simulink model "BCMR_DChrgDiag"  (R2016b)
settings: Solver=FixedStepDiscrete  StartTime=0.0  StopTime=10  FixedStep=0.01  RelTol=1e-3  EnableMultiTasking=on
undefined symbols (not defined in the file or in its folder): BCMR_bDChrgStopCActiveSw_C, BCMR_cntDChrgTCnntMax_C, BCMR_cntIsoFltTrigger_CW, BCMR_EVCCDiagccSw_C, BCMR_EVCCDiagSw_C, BCMR_G1E0PlatformSwDiag_C, BCMR_H1U0PlatformSwDiag_C, BCMR_iDcChrgDiffOvrCurr_C, BCMR_iDcChrgLowTempDiffOvrCurrMody_C, BCMR_iDcChrgLowTempOvrCurrCutOff_C, BCMR_iDcChrgLowTempOvrCurrHeal_C, BCMR_iDcChrgOvrCurr_C, BCMR_iDcChrgOvrVolt_C, BCMR_iDChrgCurrDiagLmt_C, BCMR_iDChrgCutOffVoltOvrCurrDet_C, BCMR_iDChrgCutOffVoltOvrCurrHeal_C, BCMR_kWaveFltFactor_C, BCMR_stCCSTimeout_C, BCMR_stCHMTimeout_C, BCMR_stCMLTimeout_C, BCMR_stCRMAATimeout_C, BCMR_stCROAATimeout_C, BCMR_stCROTimeout_C, BCMR_stCSDTimeout1_C, BCMR_stCSDTimeout2_C, BCMR_stCSTTimeout_C, BCMR_stCurrDwnTimeout_C, BCMR_stHvOnTimeout_C, BCMR_stNoTimeout_C, BCMR_stParaMish_C, BCMR_tBattLowTempDiagTempThrd_C, BCMR_tDcChrgIntfTempDiffLmt_C, BCMR_tDcChrgIntfTempLmt_C, BCMR_tiDChrgDetDiagDebs_C, BCMR_tiDChrgDetSec_C, BCMR_tiDChrgDiagBase_C, BCMR_tiDChrgHealDiagDebs_C, BCMR_tiDChrgIntfTempDwnLmt_C, BCMR_tiDChrgLowTOvrCurrDet_C, BCMR_tiDChrgLowTOvrCurrHeal_C, BCMR_tiDChrgMishCurrDetDiagDebs_C, BCMR_tiDChrgOvrCellVolt_C, BCMR_tiDChrgOvrSafeCellVoltDet_C, BCMR_tiDChrgVoltFltDetDebs_C, BCMR_tiDChrgVoltFltHealDebs_C, BCMR_uCC2ChkDiffDet_C, BCMR_uCC2ChkDiffHeal_C, BCMR_uCC2VoltHighDet_C, BCMR_uCC2VoltHighHeal_C, BCMR_uCC2VoltLowDet_C, BCMR_uCC2VoltLowHeal_C, BCMR_uDChrgHighTempDet_C, BCMR_uDChrgHighTempHeal_C, BCMR_uDChrgLowTempDet_C, BCMR_uDChrgLowTempHeal_C, BCMR_uDChrgOvrCellVoltDet_C, BCMR_uDChrgOvrCellVoltHeal_C, BCMR_uDChrgOvrSafeCellVoltDet_C, BCMR_uDChrgOvrSafeCellVoltHeal_C, bin2dec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
libraries: simulink x291
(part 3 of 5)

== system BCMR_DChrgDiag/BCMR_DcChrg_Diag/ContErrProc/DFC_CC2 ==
  BCMR_bDcOutputContErrDet : Inport
  BCMR_bDcOutputContErrHeal : Inport  Port=2
  BCMR_bCC2VolttLowErrDet : Inport  Port=3
  BCMR_bCC2VoltLowErrHeal : Inport  Port=4
  BCMR_bCC2VoltHighErrDet : Inport  Port=5
  BCMR_bCC2VoltHighErrHeal : Inport  Port=6
  Bitwise Operator9 : simulink/Logic and Bit Operations/Bitwise Operator  logicop=AND  UseBitMask=on  BitMask=bin2dec('00011000')  BitMaskRealWorld=Stored Integer
  Compare To Constant3 : simulink/Logic and Bit Operations/Compare To Constant  relop===  const=24  OutDataTypeStr=boolean
  DSM_ReportCheckSelfHeal : Subsystem  TreatAsAtomicUnit=on  RTWFcnName=DSM_ReportCheck  RTWFileName=SrvLib
  Data Store Read2 : DataStoreRead  DataStoreName=DFC_CC2Chk
  Data Store Read3 : DataStoreRead  DataStoreName=DFC_CC2Chk
  Data Store Write1 : DataStoreWrite  DataStoreName=DFC_CC2Chk
  Data Type Conversion1 : DataTypeConversion  OutDataTypeStr=uint8
  Logical Operator1 : Logic  Operator=OR  Inputs=3  AllPortsSameDT=off  OutDataTypeStr=boolean
  Logical Operator2 : Logic  Inputs=3  AllPortsSameDT=off  OutDataTypeStr=boolean
  BCMR_stCC2ChkVoltErr : Outport  OutputWhenDisabled=reset  InitialOutput=[0]
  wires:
  Compare To Constant3/1 -> Data Type Conversion1/1
  Bitwise Operator9/1 -> Compare To Constant3/1
  Logical Operator1/1 -> DSM_ReportCheckSelfHeal/2(Err)
  Logical Operator2/1 -> DSM_ReportCheckSelfHeal/3(Heal)
  DSM_ReportCheckSelfHeal/1(Dfc_id) -> Data Store Write1/1
  Data Store Read2/1 -> DSM_ReportCheckSelfHeal/1(Dfc_id_nv)
  Data Store Read3/1 -> Bitwise Operator9/1
  Data Type Conversion1/1 -> BCMR_stCC2ChkVoltErr/1  "BCMR_stCC2ChkVoltErr"
  BCMR_bCC2VoltHighErrHeal/1 -> Logical Operator2/3
  BCMR_bCC2VoltLowErrHeal/1 -> Logical Operator2/2
  BCMR_bDcOutputContErrHeal/1 -> Logical Operator2/1
  BCMR_bCC2VoltHighErrDet/1 -> Logical Operator1/3
  BCMR_bCC2VolttLowErrDet/1 -> Logical Operator1/2
  BCMR_bDcOutputContErrDet/1 -> Logical Operator1/1

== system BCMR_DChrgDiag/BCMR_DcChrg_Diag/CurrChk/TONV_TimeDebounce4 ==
  note: Turn On Delay Time Deboune
  T : Inport
  u : Inport  Port=2
  dT : Inport  Port=3
  Add : Sum
  Constant1 : Constant  Value=0  OutDataTypeStr=uint8
  Constant2 : Constant  OutDataTypeStr=uint8
  Constant3 : Constant  Value=0  OutDataTypeStr=single
  Delay : Delay  DelayLength=1  InitialCondition=0
  MinMax : MinMax  Inputs=2
  Product : Product  OutMin=[0]  OutMax=[65535]  OutDataTypeStr=single
  Relational Operator : RelationalOperator  OutDataTypeStr=boolean  RndMeth=Simplest
  Switch : Switch  Criteria=u2 ~= 0
  Switch1 : Switch  Criteria=u2 ~= 0
  y : Outport
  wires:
  u/1 -> Switch1/2, Switch/2
  Switch/1 -> Product/1
  dT/1 -> Switch1/1
  Constant3/1 -> Switch1/3
  Constant2/1 -> Switch/1
  Constant1/1 -> Switch/3
  Add/1 -> Product/2
  Product/1 -> Relational Operator/1, Delay/1
  Switch1/1 -> Add/1
  Delay/1 -> MinMax/2
  Relational Operator/1 -> y/1
  T/1 -> Relational Operator/2, MinMax/1
  MinMax/1 -> Add/2

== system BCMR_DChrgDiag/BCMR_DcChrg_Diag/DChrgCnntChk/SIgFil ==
  u : Inport
  Constant4 : Constant  Value=0  OutDataTypeStr=boolean
  Delay1 : Delay  DelayLength=1  InitialCondition=0
  Filter : Subsystem
  Switch4 : Switch  Criteria=u2 ~= 0
  Unit Delay1 : UnitDelay  InitialCondition=1  SampleTime=-1
  y : Outport
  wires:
  Delay1/1 -> Filter/2(In2)
  u/1 -> Filter/1(In1), Switch4/1
  Unit Delay1/1 -> Switch4/2
  Constant4/1 -> Unit Delay1/1
  Filter/1(Out) -> Switch4/3
  Switch4/1 -> y/1, Delay1/1

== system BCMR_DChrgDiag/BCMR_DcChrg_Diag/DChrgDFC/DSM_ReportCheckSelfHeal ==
  note: Fault report to diagnostic management system
  Dfc_id_nv : Inport  OutDataTypeStr=uint8
  Err : Inport  Port=2
  Heal : Inport  Port=3
  Bit Clear1 : simulink/Logic and Bit Operations/Bit Clear  iBit=4
  Bit Clear2 : simulink/Logic and Bit Operations/Bit Clear  iBit=3
  Bit Set : simulink/Logic and Bit Operations/Bit Set  iBit=4
  Bit Set1 : simulink/Logic and Bit Operations/Bit Set  iBit=3
  Bit Set2 : simulink/Logic and Bit Operations/Bit Set  iBit=3
  Bit Set4 : simulink/Logic and Bit Operations/Bit Set  iBit=7
  Constant1 : Constant  Value=0  OutDataTypeStr=uint8
  Constant7 : Constant  Value=0  OutDataTypeStr=boolean
  Delay2 : Delay  DelayLength=1  InitialCondition=1
  Delay3 : Delay  DelayLength=1  InitialCondition=0
  Logical Operator : Logic  Operator=OR  AllPortsSameDT=off  OutDataTypeStr=boolean
  Switch{1..4} (4 alike) : Switch  Criteria=u2 ~= 0
  Dfc_id : Outport  OutDataTypeStr=uint8
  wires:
  Dfc_id_nv/1 -> Bit Clear2/1, Bit Set4/1, Bit Clear1/1
  Bit Set4/1 -> Bit Set/1
  Constant7/1 -> Delay2/1
  Delay2/1 -> Switch2/2
  Switch3/1 -> Switch2/3
  Bit Clear2/1 -> Switch2/1
  Switch2/1 -> Delay3/1, Switch1/1
  Bit Set1/1 -> Switch3/1
  Bit Set/1 -> Bit Set1/1
  Switch4/1 -> Switch3/3
  Err/1 -> Logical Operator/2, Switch3/2
  Bit Set2/1 -> Switch4/1
  Bit Clear1/1 -> Bit Set2/1
  Delay3/1 -> Switch4/3
  Heal/1 -> Logical Operator/1, Switch4/2
  Logical Operator/1 -> Switch1/2
  Constant1/1 -> Switch1/3
  Switch1/1 -> Dfc_id/1

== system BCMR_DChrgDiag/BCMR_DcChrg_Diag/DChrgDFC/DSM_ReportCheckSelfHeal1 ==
  note: Fault report to diagnostic management system
  Dfc_id_nv : Inport  OutDataTypeStr=uint8
  Err : Inport  Port=2
  Heal : Inport  Port=3
  Bit Clear1 : simulink/Logic and Bit Operations/Bit Clear  iBit=4
  Bit Clear2 : simulink/Logic and Bit Operations/Bit Clear  iBit=3
  Bit Set : simulink/Logic and Bit Operations/Bit Set  iBit=4
  Bit Set1 : simulink/Logic and Bit Operations/Bit Set  iBit=3
  Bit Set2 : simulink/Logic and Bit Operations/Bit Set  iBit=3
  Bit Set4 : simulink/Logic and Bit Operations/Bit Set  iBit=7
  Constant1 : Constant  Value=0  OutDataTypeStr=uint8
  Constant7 : Constant  Value=0  OutDataTypeStr=boolean
  Delay2 : Delay  DelayLength=1  InitialCondition=1
  Delay3 : Delay  DelayLength=1  InitialCondition=0
  Logical Operator : Logic  Operator=OR  AllPortsSameDT=off  OutDataTypeStr=boolean
  Switch{1..4} (4 alike) : Switch  Criteria=u2 ~= 0
  Dfc_id : Outport  OutDataTypeStr=uint8
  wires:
  Dfc_id_nv/1 -> Bit Clear2/1, Bit Set4/1, Bit Clear1/1
  Bit Set4/1 -> Bit Set/1
  Constant7/1 -> Delay2/1
  Delay2/1 -> Switch2/2
  Switch3/1 -> Switch2/3
  Bit Clear2/1 -> Switch2/1
  Switch2/1 -> Delay3/1, Switch1/1
  Bit Set1/1 -> Switch3/1
  Bit Set/1 -> Bit Set1/1
  Switch4/1 -> Switch3/3
  Err/1 -> Logical Operator/2, Switch3/2
  Bit Set2/1 -> Switch4/1
  Bit Clear1/1 -> Bit Set2/1
  Delay3/1 -> Switch4/3
  Heal/1 -> Logical Operator/1, Switch4/2
  Logical Operator/1 -> Switch1/2
  Constant1/1 -> Switch1/3
  Switch1/1 -> Dfc_id/1

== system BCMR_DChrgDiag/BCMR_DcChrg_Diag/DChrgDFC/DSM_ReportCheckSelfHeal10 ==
  note: Fault report to diagnostic management system
  Dfc_id_nv : Inport  OutDataTypeStr=uint8
  Err : Inport  Port=2
  Heal : Inport  Port=3
  Bit Clear1 : simulink/Logic and Bit Operations/Bit Clear  iBit=4
  Bit Clear2 : simulink/Logic and Bit Operations/Bit Clear  iBit=3
  Bit Set : simulink/Logic and Bit Operations/Bit Set  iBit=4
  Bit Set1 : simulink/Logic and Bit Operations/Bit Set  iBit=3
  Bit Set2 : simulink/Logic and Bit Operations/Bit Set  iBit=3
  Bit Set4 : simulink/Logic and Bit Operations/Bit Set  iBit=7
  Constant1 : Constant  Value=0  OutDataTypeStr=uint8
  Constant7 : Constant  Value=0  OutDataTypeStr=boolean
  Delay2 : Delay  DelayLength=1  InitialCondition=1
  Delay3 : Delay  DelayLength=1  InitialCondition=0
  Logical Operator : Logic  Operator=OR  AllPortsSameDT=off  OutDataTypeStr=boolean
  Switch{1..4} (4 alike) : Switch  Criteria=u2 ~= 0
  Dfc_id : Outport  OutDataTypeStr=uint8
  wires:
  Dfc_id_nv/1 -> Bit Clear2/1, Bit Set4/1, Bit Clear1/1
  Bit Set4/1 -> Bit Set/1
  Constant7/1 -> Delay2/1
  Delay2/1 -> Switch2/2
  Switch3/1 -> Switch2/3
  Bit Clear2/1 -> Switch2/1
  Switch2/1 -> Delay3/1, Switch1/1
  Bit Set1/1 -> Switch3/1
  Bit Set/1 -> Bit Set1/1
  Switch4/1 -> Switch3/3
  Err/1 -> Logical Operator/2, Switch3/2
  Bit Set2/1 -> Switch4/1
  Bit Clear1/1 -> Bit Set2/1
  Delay3/1 -> Switch4/3
  Heal/1 -> Logical Operator/1, Switch4/2
  Logical Operator/1 -> Switch1/2
  Constant1/1 -> Switch1/3
  Switch1/1 -> Dfc_id/1

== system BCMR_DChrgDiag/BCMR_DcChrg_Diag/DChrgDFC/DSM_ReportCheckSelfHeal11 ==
  note: Fault report to diagnostic management system
  Dfc_id_nv : Inport  OutDataTypeStr=uint8
  Err : Inport  Port=2
  Heal : Inport  Port=3
  Bit Clear1 : simulink/Logic and Bit Operations/Bit Clear  iBit=4
  Bit Clear2 : simulink/Logic and Bit Operations/Bit Clear  iBit=3
  Bit Set : simulink/Logic and Bit Operations/Bit Set  iBit=4
  Bit Set1 : simulink/Logic and Bit Operations/Bit Set  iBit=3
  Bit Set2 : simulink/Logic and Bit Operations/Bit Set  iBit=3
  Bit Set4 : simulink/Logic and Bit Operations/Bit Set  iBit=7
  Constant1 : Constant  Value=0  OutDataTypeStr=uint8
  Constant7 : Constant  Value=0  OutDataTypeStr=boolean
  Delay2 : Delay  DelayLength=1  InitialCondition=1
  Delay3 : Delay  DelayLength=1  InitialCondition=0
  Logical Operator : Logic  Operator=OR  AllPortsSameDT=off  OutDataTypeStr=boolean
  Switch{1..4} (4 alike) : Switch  Criteria=u2 ~= 0
  Dfc_id : Outport  OutDataTypeStr=uint8
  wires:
  Dfc_id_nv/1 -> Bit Clear2/1, Bit Set4/1, Bit Clear1/1
  Bit Set4/1 -> Bit Set/1
  Constant7/1 -> Delay2/1
  Delay2/1 -> Switch2/2
  Switch3/1 -> Switch2/3
  Bit Clear2/1 -> Switch2/1
  Switch2/1 -> Delay3/1, Switch1/1
  Bit Set1/1 -> Switch3/1
  Bit Set/1 -> Bit Set1/1
  Switch4/1 -> Switch3/3
  Err/1 -> Logical Operator/2, Switch3/2
  Bit Set2/1 -> Switch4/1
  Bit Clear1/1 -> Bit Set2/1
  Delay3/1 -> Switch4/3
  Heal/1 -> Logical Operator/1, Switch4/2
  Logical Operator/1 -> Switch1/2
  Constant1/1 -> Switch1/3
  Switch1/1 -> Dfc_id/1

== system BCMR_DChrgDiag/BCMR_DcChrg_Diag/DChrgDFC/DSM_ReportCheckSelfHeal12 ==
  note: Fault report to diagnostic management system
  Dfc_id_nv : Inport  OutDataTypeStr=uint8
  Err : Inport  Port=2
  Heal : Inport  Port=3
  Bit Clear1 : simulink/Logic and Bit Operations/Bit Clear  iBit=4
  Bit Clear2 : simulink/Logic and Bit Operations/Bit Clear  iBit=3
  Bit Set : simulink/Logic and Bit Operations/Bit Set  iBit=4
  Bit Set1 : simulink/Logic and Bit Operations/Bit Set  iBit=3
  Bit Set2 : simulink/Logic and Bit Operations/Bit Set  iBit=3
  Bit Set4 : simulink/Logic and Bit Operations/Bit Set  iBit=7
  Constant1 : Constant  Value=0  OutDataTypeStr=uint8
  Constant7 : Constant  Value=0  OutDataTypeStr=boolean
  Delay2 : Delay  DelayLength=1  InitialCondition=1
  Delay3 : Delay  DelayLength=1  InitialCondition=0
  Logical Operator : Logic  Operator=OR  AllPortsSameDT=off  OutDataTypeStr=boolean
  Switch{1..4} (4 alike) : Switch  Criteria=u2 ~= 0
  Dfc_id : Outport  OutDataTypeStr=uint8
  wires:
  Dfc_id_nv/1 -> Bit Clear2/1, Bit Set4/1, Bit Clear1/1
  Bit Set4/1 -> Bit Set/1
  Constant7/1 -> Delay2/1
  Delay2/1 -> Switch2/2
  Switch3/1 -> Switch2/3
  Bit Clear2/1 -> Switch2/1
  Switch2/1 -> Delay3/1, Switch1/1
  Bit Set1/1 -> Switch3/1
  Bit Set/1 -> Bit Set1/1
  Switch4/1 -> Switch3/3
  Err/1 -> Logical Operator/2, Switch3/2
  Bit Set2/1 -> Switch4/1
  Bit Clear1/1 -> Bit Set2/1
  Delay3/1 -> Switch4/3
  Heal/1 -> Logical Operator/1, Switch4/2
  Logical Operator/1 -> Switch1/2
  Constant1/1 -> Switch1/3
  Switch1/1 -> Dfc_id/1

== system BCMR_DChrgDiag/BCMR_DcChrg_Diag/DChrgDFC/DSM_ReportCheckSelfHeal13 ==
  note: Fault report to diagnostic management system
  Dfc_id_nv : Inport  OutDataTypeStr=uint8
  Err : Inport  Port=2
  Heal : Inport  Port=3
  Bit Clear1 : simulink/Logic and Bit Operations/Bit Clear  iBit=4
  Bit Clear2 : simulink/Logic and Bit Operations/Bit Clear  iBit=3
  Bit Set : simulink/Logic and Bit Operations/Bit Set  iBit=4
  Bit Set1 : simulink/Logic and Bit Operations/Bit Set  iBit=3
  Bit Set2 : simulink/Logic and Bit Operations/Bit Set  iBit=3
  Bit Set4 : simulink/Logic and Bit Operations/Bit Set  iBit=7
  Constant1 : Constant  Value=0  OutDataTypeStr=uint8
  Constant7 : Constant  Value=0  OutDataTypeStr=boolean
  Delay2 : Delay  DelayLength=1  InitialCondition=1
  Delay3 : Delay  DelayLength=1  InitialCondition=0
  Logical Operator : Logic  Operator=OR  AllPortsSameDT=off  OutDataTypeStr=boolean
  Switch{1..4} (4 alike) : Switch  Criteria=u2 ~= 0
  Dfc_id : Outport  OutDataTypeStr=uint8
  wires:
  Dfc_id_nv/1 -> Bit Clear2/1, Bit Set4/1, Bit Clear1/1
  Bit Set4/1 -> Bit Set/1
  Constant7/1 -> Delay2/1
  Delay2/1 -> Switch2/2
  Switch3/1 -> Switch2/3
  Bit Clear2/1 -> Switch2/1
  Switch2/1 -> Delay3/1, Switch1/1
  Bit Set1/1 -> Switch3/1
  Bit Set/1 -> Bit Set1/1
  Switch4/1 -> Switch3/3
  Err/1 -> Logical Operator/2, Switch3/2
  Bit Set2/1 -> Switch4/1
  Bit Clear1/1 -> Bit Set2/1
  Delay3/1 -> Switch4/3
  Heal/1 -> Logical Operator/1, Switch4/2
  Logical Operator/1 -> Switch1/2
  Constant1/1 -> Switch1/3
  Switch1/1 -> Dfc_id/1

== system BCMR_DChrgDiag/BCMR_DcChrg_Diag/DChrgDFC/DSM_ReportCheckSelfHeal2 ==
  note: Fault report to diagnostic management system
  Dfc_id_nv : Inport  OutDataTypeStr=uint8
  Err : Inport  Port=2
  Heal : Inport  Port=3
  Bit Clear1 : simulink/Logic and Bit Operations/Bit Clear  iBit=4
  Bit Clear2 : simulink/Logic and Bit Operations/Bit Clear  iBit=3
  Bit Set : simulink/Logic and Bit Operations/Bit Set  iBit=4
  Bit Set1 : simulink/Logic and Bit Operations/Bit Set  iBit=3
  Bit Set2 : simulink/Logic and Bit Operations/Bit Set  iBit=3
  Bit Set4 : simulink/Logic and Bit Operations/Bit Set  iBit=7
  Constant1 : Constant  Value=0  OutDataTypeStr=uint8
  Constant7 : Constant  Value=0  OutDataTypeStr=boolean
  Delay2 : Delay  DelayLength=1  InitialCondition=1
  Delay3 : Delay  DelayLength=1  InitialCondition=0
  Logical Operator : Logic  Operator=OR  AllPortsSameDT=off  OutDataTypeStr=boolean
  Switch{1..4} (4 alike) : Switch  Criteria=u2 ~= 0
  Dfc_id : Outport  OutDataTypeStr=uint8
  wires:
  Dfc_id_nv/1 -> Bit Clear2/1, Bit Set4/1, Bit Clear1/1
  Bit Set4/1 -> Bit Set/1
  Constant7/1 -> Delay2/1
  Delay2/1 -> Switch2/2
  Switch3/1 -> Switch2/3
  Bit Clear2/1 -> Switch2/1
  Switch2/1 -> Delay3/1, Switch1/1
  Bit Set1/1 -> Switch3/1
  Bit Set/1 -> Bit Set1/1
  Switch4/1 -> Switch3/3
  Err/1 -> Logical Operator/2, Switch3/2
  Bit Set2/1 -> Switch4/1
  Bit Clear1/1 -> Bit Set2/1
  Delay3/1 -> Switch4/3
  Heal/1 -> Logical Operator/1, Switch4/2
  Logical Operator/1 -> Switch1/2
  Constant1/1 -> Switch1/3
  Switch1/1 -> Dfc_id/1

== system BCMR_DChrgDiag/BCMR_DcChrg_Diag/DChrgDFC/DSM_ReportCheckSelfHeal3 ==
  note: Fault report to diagnostic management system
  Dfc_id_nv : Inport  OutDataTypeStr=uint8
  Err : Inport  Port=2
  Heal : Inport  Port=3
  Bit Clear1 : simulink/Logic and Bit Operations/Bit Clear  iBit=4
  Bit Clear2 : simulink/Logic and Bit Operations/Bit Clear  iBit=3
  Bit Set : simulink/Logic and Bit Operations/Bit Set  iBit=4
  Bit Set1 : simulink/Logic and Bit Operations/Bit Set  iBit=3
  Bit Set2 : simulink/Logic and Bit Operations/Bit Set  iBit=3
  Bit Set4 : simulink/Logic and Bit Operations/Bit Set  iBit=7
  Constant1 : Constant  Value=0  OutDataTypeStr=uint8
  Constant7 : Constant  Value=0  OutDataTypeStr=boolean
  Delay2 : Delay  DelayLength=1  InitialCondition=1
  Delay3 : Delay  DelayLength=1  InitialCondition=0
  Logical Operator : Logic  Operator=OR  AllPortsSameDT=off  OutDataTypeStr=boolean
  Switch{1..4} (4 alike) : Switch  Criteria=u2 ~= 0
  Dfc_id : Outport  OutDataTypeStr=uint8
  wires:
  Dfc_id_nv/1 -> Bit Clear2/1, Bit Set4/1, Bit Clear1/1
  Bit Set4/1 -> Bit Set/1
  Constant7/1 -> Delay2/1
  Delay2/1 -> Switch2/2
  Switch3/1 -> Switch2/3
  Bit Clear2/1 -> Switch2/1
  Switch2/1 -> Delay3/1, Switch1/1
  Bit Set1/1 -> Switch3/1
  Bit Set/1 -> Bit Set1/1
  Switch4/1 -> Switch3/3
  Err/1 -> Logical Operator/2, Switch3/2
  Bit Set2/1 -> Switch4/1
  Bit Clear1/1 -> Bit Set2/1
  Delay3/1 -> Switch4/3
  Heal/1 -> Logical Operator/1, Switch4/2
  Logical Operator/1 -> Switch1/2
  Constant1/1 -> Switch1/3
  Switch1/1 -> Dfc_id/1

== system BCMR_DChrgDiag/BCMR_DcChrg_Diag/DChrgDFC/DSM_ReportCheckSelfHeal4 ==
  note: Fault report to diagnostic management system
  Dfc_id_nv : Inport  OutDataTypeStr=uint8
  Err : Inport  Port=2
  Heal : Inport  Port=3
  Bit Clear1 : simulink/Logic and Bit Operations/Bit Clear  iBit=4
  Bit Clear2 : simulink/Logic and Bit Operations/Bit Clear  iBit=3
  Bit Set : simulink/Logic and Bit Operations/Bit Set  iBit=4
  Bit Set1 : simulink/Logic and Bit Operations/Bit Set  iBit=3
  Bit Set2 : simulink/Logic and Bit Operations/Bit Set  iBit=3
  Bit Set4 : simulink/Logic and Bit Operations/Bit Set  iBit=7
  Constant1 : Constant  Value=0  OutDataTypeStr=uint8
  Constant7 : Constant  Value=0  OutDataTypeStr=boolean
  Delay2 : Delay  DelayLength=1  InitialCondition=1
  Delay3 : Delay  DelayLength=1  InitialCondition=0
  Logical Operator : Logic  Operator=OR  AllPortsSameDT=off  OutDataTypeStr=boolean
  Switch{1..4} (4 alike) : Switch  Criteria=u2 ~= 0
  Dfc_id : Outport  OutDataTypeStr=uint8
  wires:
  Dfc_id_nv/1 -> Bit Clear2/1, Bit Set4/1, Bit Clear1/1
  Bit Set4/1 -> Bit Set/1
  Constant7/1 -> Delay2/1
  Delay2/1 -> Switch2/2
  Switch3/1 -> Switch2/3
  Bit Clear2/1 -> Switch2/1
  Switch2/1 -> Delay3/1, Switch1/1
  Bit Set1/1 -> Switch3/1
  Bit Set/1 -> Bit Set1/1
  Switch4/1 -> Switch3/3
  Err/1 -> Logical Operator/2, Switch3/2
  Bit Set2/1 -> Switch4/1
  Bit Clear1/1 -> Bit Set2/1
  Delay3/1 -> Switch4/3
  Heal/1 -> Logical Operator/1, Switch4/2
  Logical Operator/1 -> Switch1/2
  Constant1/1 -> Switch1/3
  Switch1/1 -> Dfc_id/1

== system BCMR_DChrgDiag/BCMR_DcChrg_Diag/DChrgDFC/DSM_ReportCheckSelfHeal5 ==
  note: Fault report to diagnostic management system
  Dfc_id_nv : Inport  OutDataTypeStr=uint8
  Err : Inport  Port=2
  Heal : Inport  Port=3
  Bit Clear1 : simulink/Logic and Bit Operations/Bit Clear  iBit=4
  Bit Clear2 : simulink/Logic and Bit Operations/Bit Clear  iBit=3
  Bit Set : simulink/Logic and Bit Operations/Bit Set  iBit=4
  Bit Set1 : simulink/Logic and Bit Operations/Bit Set  iBit=3
  Bit Set2 : simulink/Logic and Bit Operations/Bit Set  iBit=3
  Bit Set4 : simulink/Logic and Bit Operations/Bit Set  iBit=7
  Constant1 : Constant  Value=0  OutDataTypeStr=uint8
  Constant7 : Constant  Value=0  OutDataTypeStr=boolean
  Delay2 : Delay  DelayLength=1  InitialCondition=1
  Delay3 : Delay  DelayLength=1  InitialCondition=0
  Logical Operator : Logic  Operator=OR  AllPortsSameDT=off  OutDataTypeStr=boolean
  Switch{1..4} (4 alike) : Switch  Criteria=u2 ~= 0
  Dfc_id : Outport  OutDataTypeStr=uint8
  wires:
  Dfc_id_nv/1 -> Bit Clear2/1, Bit Set4/1, Bit Clear1/1
  Bit Set4/1 -> Bit Set/1
  Constant7/1 -> Delay2/1
  Delay2/1 -> Switch2/2
  Switch3/1 -> Switch2/3
  Bit Clear2/1 -> Switch2/1
  Switch2/1 -> Delay3/1, Switch1/1
  Bit Set1/1 -> Switch3/1
  Bit Set/1 -> Bit Set1/1
  Switch4/1 -> Switch3/3
  Err/1 -> Logical Operator/2, Switch3/2
  Bit Set2/1 -> Switch4/1
  Bit Clear1/1 -> Bit Set2/1
  Delay3/1 -> Switch4/3
  Heal/1 -> Logical Operator/1, Switch4/2
  Logical Operator/1 -> Switch1/2
  Constant1/1 -> Switch1/3
  Switch1/1 -> Dfc_id/1

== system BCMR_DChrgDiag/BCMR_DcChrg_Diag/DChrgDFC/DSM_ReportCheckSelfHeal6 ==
  note: Fault report to diagnostic management system
  Dfc_id_nv : Inport  OutDataTypeStr=uint8
  Err : Inport  Port=2
  Heal : Inport  Port=3
  Bit Clear1 : simulink/Logic and Bit Operations/Bit Clear  iBit=4
  Bit Clear2 : simulink/Logic and Bit Operations/Bit Clear  iBit=3
  Bit Set : simulink/Logic and Bit Operations/Bit Set  iBit=4
  Bit Set1 : simulink/Logic and Bit Operations/Bit Set  iBit=3
  Bit Set2 : simulink/Logic and Bit Operations/Bit Set  iBit=3
  Bit Set4 : simulink/Logic and Bit Operations/Bit Set  iBit=7
  Constant1 : Constant  Value=0  OutDataTypeStr=uint8
  Constant7 : Constant  Value=0  OutDataTypeStr=boolean
  Delay2 : Delay  DelayLength=1  InitialCondition=1
  Delay3 : Delay  DelayLength=1  InitialCondition=0
  Logical Operator : Logic  Operator=OR  AllPortsSameDT=off  OutDataTypeStr=boolean
  Switch{1..4} (4 alike) : Switch  Criteria=u2 ~= 0
  Dfc_id : Outport  OutDataTypeStr=uint8
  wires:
  Dfc_id_nv/1 -> Bit Clear2/1, Bit Set4/1, Bit Clear1/1
  Bit Set4/1 -> Bit Set/1
  Constant7/1 -> Delay2/1
  Delay2/1 -> Switch2/2
  Switch3/1 -> Switch2/3
  Bit Clear2/1 -> Switch2/1
  Switch2/1 -> Delay3/1, Switch1/1
  Bit Set1/1 -> Switch3/1
  Bit Set/1 -> Bit Set1/1
  Switch4/1 -> Switch3/3
  Err/1 -> Logical Operator/2, Switch3/2
  Bit Set2/1 -> Switch4/1
  Bit Clear1/1 -> Bit Set2/1
  Delay3/1 -> Switch4/3
  Heal/1 -> Logical Operator/1, Switch4/2
  Logical Operator/1 -> Switch1/2
  Constant1/1 -> Switch1/3
  Switch1/1 -> Dfc_id/1

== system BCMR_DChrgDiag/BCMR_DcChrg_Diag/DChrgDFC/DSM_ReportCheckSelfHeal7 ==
  note: Fault report to diagnostic management system
  Dfc_id_nv : Inport  OutDataTypeStr=uint8
  Err : Inport  Port=2
  Heal : Inport  Port=3
  Bit Clear1 : simulink/Logic and Bit Operations/Bit Clear  iBit=4
  Bit Clear2 : simulink/Logic and Bit Operations/Bit Clear  iBit=3
  Bit Set : simulink/Logic and Bit Operations/Bit Set  iBit=4
  Bit Set1 : simulink/Logic and Bit Operations/Bit Set  iBit=3
  Bit Set2 : simulink/Logic and Bit Operations/Bit Set  iBit=3
  Bit Set4 : simulink/Logic and Bit Operations/Bit Set  iBit=7
  Constant1 : Constant  Value=0  OutDataTypeStr=uint8
  Constant7 : Constant  Value=0  OutDataTypeStr=boolean
  Delay2 : Delay  DelayLength=1  InitialCondition=1
  Delay3 : Delay  DelayLength=1  InitialCondition=0
  Logical Operator : Logic  Operator=OR  AllPortsSameDT=off  OutDataTypeStr=boolean
  Switch{1..4} (4 alike) : Switch  Criteria=u2 ~= 0
  Dfc_id : Outport  OutDataTypeStr=uint8
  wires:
  Dfc_id_nv/1 -> Bit Clear2/1, Bit Set4/1, Bit Clear1/1
  Bit Set4/1 -> Bit Set/1
  Constant7/1 -> Delay2/1
  Delay2/1 -> Switch2/2
  Switch3/1 -> Switch2/3
  Bit Clear2/1 -> Switch2/1
  Switch2/1 -> Delay3/1, Switch1/1
  Bit Set1/1 -> Switch3/1
  Bit Set/1 -> Bit Set1/1
  Switch4/1 -> Switch3/3
  Err/1 -> Logical Operator/2, Switch3/2
  Bit Set2/1 -> Switch4/1
  Bit Clear1/1 -> Bit Set2/1
  Delay3/1 -> Switch4/3
  Heal/1 -> Logical Operator/1, Switch4/2
  Logical Operator/1 -> Switch1/2
  Constant1/1 -> Switch1/3
  Switch1/1 -> Dfc_id/1

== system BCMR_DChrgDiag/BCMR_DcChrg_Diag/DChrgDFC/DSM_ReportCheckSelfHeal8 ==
  note: Fault report to diagnostic management system
  Dfc_id_nv : Inport  OutDataTypeStr=uint8
  Err : Inport  Port=2
  Heal : Inport  Port=3
  Bit Clear1 : simulink/Logic and Bit Operations/Bit Clear  iBit=4
  Bit Clear2 : simulink/Logic and Bit Operations/Bit Clear  iBit=3
  Bit Set : simulink/Logic and Bit Operations/Bit Set  iBit=4
  Bit Set1 : simulink/Logic and Bit Operations/Bit Set  iBit=3
  Bit Set2 : simulink/Logic and Bit Operations/Bit Set  iBit=3
  Bit Set4 : simulink/Logic and Bit Operations/Bit Set  iBit=7
  Constant1 : Constant  Value=0  OutDataTypeStr=uint8
  Constant7 : Constant  Value=0  OutDataTypeStr=boolean
  Delay2 : Delay  DelayLength=1  InitialCondition=1
  Delay3 : Delay  DelayLength=1  InitialCondition=0
  Logical Operator : Logic  Operator=OR  AllPortsSameDT=off  OutDataTypeStr=boolean
  Switch{1..4} (4 alike) : Switch  Criteria=u2 ~= 0
  Dfc_id : Outport  OutDataTypeStr=uint8
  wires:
  Dfc_id_nv/1 -> Bit Clear2/1, Bit Set4/1, Bit Clear1/1
  Bit Set4/1 -> Bit Set/1
  Constant7/1 -> Delay2/1
  Delay2/1 -> Switch2/2
  Switch3/1 -> Switch2/3
  Bit Clear2/1 -> Switch2/1
  Switch2/1 -> Delay3/1, Switch1/1
  Bit Set1/1 -> Switch3/1
  Bit Set/1 -> Bit Set1/1
  Switch4/1 -> Switch3/3
  Err/1 -> Logical Operator/2, Switch3/2
  Bit Set2/1 -> Switch4/1
  Bit Clear1/1 -> Bit Set2/1
  Delay3/1 -> Switch4/3
  Heal/1 -> Logical Operator/1, Switch4/2
  Logical Operator/1 -> Switch1/2
  Constant1/1 -> Switch1/3
  Switch1/1 -> Dfc_id/1

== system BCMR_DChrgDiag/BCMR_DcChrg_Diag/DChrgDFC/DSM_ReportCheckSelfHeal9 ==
  note: Fault report to diagnostic management system
  Dfc_id_nv : Inport  OutDataTypeStr=uint8
  Err : Inport  Port=2
  Heal : Inport  Port=3
  Bit Clear1 : simulink/Logic and Bit Operations/Bit Clear  iBit=4
  Bit Clear2 : simulink/Logic and Bit Operations/Bit Clear  iBit=3
  Bit Set : simulink/Logic and Bit Operations/Bit Set  iBit=4
  Bit Set1 : simulink/Logic and Bit Operations/Bit Set  iBit=3
  Bit Set2 : simulink/Logic and Bit Operations/Bit Set  iBit=3
  Bit Set4 : simulink/Logic and Bit Operations/Bit Set  iBit=7
  Constant1 : Constant  Value=0  OutDataTypeStr=uint8
  Constant7 : Constant  Value=0  OutDataTypeStr=boolean
  Delay2 : Delay  DelayLength=1  InitialCondition=1
  Delay3 : Delay  DelayLength=1  InitialCondition=0
  Logical Operator : Logic  Operator=OR  AllPortsSameDT=off  OutDataTypeStr=boolean
  Switch{1..4} (4 alike) : Switch  Criteria=u2 ~= 0
  Dfc_id : Outport  OutDataTypeStr=uint8
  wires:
  Dfc_id_nv/1 -> Bit Clear2/1, Bit Set4/1, Bit Clear1/1
  Bit Set4/1 -> Bit Set/1
  Constant7/1 -> Delay2/1
  Delay2/1 -> Switch2/2
  Switch3/1 -> Switch2/3
  Bit Clear2/1 -> Switch2/1
  Switch2/1 -> Delay3/1, Switch1/1
  Bit Set1/1 -> Switch3/1
  Bit Set/1 -> Bit Set1/1
  Switch4/1 -> Switch3/3
  Err/1 -> Logical Operator/2, Switch3/2
  Bit Set2/1 -> Switch4/1
  Bit Clear1/1 -> Bit Set2/1
  Delay3/1 -> Switch4/3
  Heal/1 -> Logical Operator/1, Switch4/2
  Logical Operator/1 -> Switch1/2
  Constant1/1 -> Switch1/3
  Switch1/1 -> Dfc_id/1

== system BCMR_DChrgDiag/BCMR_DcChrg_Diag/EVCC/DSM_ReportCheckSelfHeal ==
  note: Fault report to diagnostic management system
  Dfc_id_nv : Inport  OutDataTypeStr=uint8
  Err : Inport  Port=2
  Heal : Inport  Port=3
  Bit Clear1 : simulink/Logic and Bit Operations/Bit Clear  iBit=4
  Bit Clear2 : simulink/Logic and Bit Operations/Bit Clear  iBit=3
  Bit Set : simulink/Logic and Bit Operations/Bit Set  iBit=4
  Bit Set1 : simulink/Logic and Bit Operations/Bit Set  iBit=3
  Bit Set2 : simulink/Logic and Bit Operations/Bit Set  iBit=3
  Bit Set4 : simulink/Logic and Bit Operations/Bit Set  iBit=7
  Constant1 : Constant  Value=0  OutDataTypeStr=uint8
  Constant7 : Constant  Value=0  OutDataTypeStr=boolean
  Delay2 : Delay  DelayLength=1  InitialCondition=1
  Delay3 : Delay  DelayLength=1  InitialCondition=0
  Logical Operator : Logic  Operator=OR  AllPortsSameDT=off  OutDataTypeStr=boolean
  Switch{1..4} (4 alike) : Switch  Criteria=u2 ~= 0
  Dfc_id : Outport  OutDataTypeStr=uint8
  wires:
  Dfc_id_nv/1 -> Bit Clear2/1, Bit Set4/1, Bit Clear1/1
  Bit Set4/1 -> Bit Set/1
  Constant7/1 -> Delay2/1
  Delay2/1 -> Switch2/2
  Switch3/1 -> Switch2/3
  Bit Clear2/1 -> Switch2/1
  Switch2/1 -> Delay3/1, Switch1/1
  Bit Set1/1 -> Switch3/1
  Bit Set/1 -> Bit Set1/1
  Switch4/1 -> Switch3/3
  Err/1 -> Logical Operator/2, Switch3/2
  Bit Set2/1 -> Switch4/1
  Bit Clear1/1 -> Bit Set2/1
  Delay3/1 -> Switch4/3
  Heal/1 -> Logical Operator/1, Switch4/2
  Logical Operator/1 -> Switch1/2
  Constant1/1 -> Switch1/3
  Switch1/1 -> Dfc_id/1

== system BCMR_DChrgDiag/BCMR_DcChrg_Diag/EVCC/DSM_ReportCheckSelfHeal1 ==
  note: Fault report to diagnostic management system
  Dfc_id_nv : Inport  OutDataTypeStr=uint8
  Err : Inport  Port=2
  Heal : Inport  Port=3
  Bit Clear1 : simulink/Logic and Bit Operations/Bit Clear  iBit=4
  Bit Clear2 : simulink/Logic and Bit Operations/Bit Clear  iBit=3
  Bit Set : simulink/Logic and Bit Operations/Bit Set  iBit=4
  Bit Set1 : simulink/Logic and Bit Operations/Bit Set  iBit=3
  Bit Set2 : simulink/Logic and Bit Operations/Bit Set  iBit=3
  Bit Set4 : simulink/Logic and Bit Operations/Bit Set  iBit=7
  Constant1 : Constant  Value=0  OutDataTypeStr=uint8
  Constant7 : Constant  Value=0  OutDataTypeStr=boolean
  Delay2 : Delay  DelayLength=1  InitialCondition=1
  Delay3 : Delay  DelayLength=1  InitialCondition=0
  Logical Operator : Logic  Operator=OR  AllPortsSameDT=off  OutDataTypeStr=boolean
  Switch{1..4} (4 alike) : Switch  Criteria=u2 ~= 0
  Dfc_id : Outport  OutDataTypeStr=uint8
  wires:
  Switch1/1 -> Dfc_id/1
  Constant1/1 -> Switch1/3
  Logical Operator/1 -> Switch1/2
  Heal/1 -> Switch4/2, Logical Operator/1
  Delay3/1 -> Switch4/3
  Bit Clear1/1 -> Bit Set2/1
  Bit Set2/1 -> Switch4/1
  Err/1 -> Switch3/2, Logical Operator/2
  Switch4/1 -> Switch3/3
  Bit Set/1 -> Bit Set1/1
  Bit Set1/1 -> Switch3/1
  Switch2/1 -> Switch1/1, Delay3/1
  Bit Clear2/1 -> Switch2/1
  Switch3/1 -> Switch2/3
  Delay2/1 -> Switch2/2
  Constant7/1 -> Delay2/1
  Bit Set4/1 -> Bit Set/1
  Dfc_id_nv/1 -> Bit Clear1/1, Bit Set4/1, Bit Clear2/1

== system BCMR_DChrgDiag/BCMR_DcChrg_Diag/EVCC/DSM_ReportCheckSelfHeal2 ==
  note: Fault report to diagnostic management system
  Dfc_id_nv : Inport  OutDataTypeStr=uint8
  Err : Inport  Port=2
  Heal : Inport  Port=3
  Bit Clear1 : simulink/Logic and Bit Operations/Bit Clear  iBit=4
  Bit Clear2 : simulink/Logic and Bit Operations/Bit Clear  iBit=3
  Bit Set : simulink/Logic and Bit Operations/Bit Set  iBit=4
  Bit Set1 : simulink/Logic and Bit Operations/Bit Set  iBit=3
  Bit Set2 : simulink/Logic and Bit Operations/Bit Set  iBit=3
  Bit Set4 : simulink/Logic and Bit Operations/Bit Set  iBit=7
  Constant1 : Constant  Value=0  OutDataTypeStr=uint8
  Constant7 : Constant  Value=0  OutDataTypeStr=boolean
  Delay2 : Delay  DelayLength=1  InitialCondition=1
  Delay3 : Delay  DelayLength=1  InitialCondition=0
  Logical Operator : Logic  Operator=OR  AllPortsSameDT=off  OutDataTypeStr=boolean
  Switch{1..4} (4 alike) : Switch  Criteria=u2 ~= 0
  Dfc_id : Outport  OutDataTypeStr=uint8
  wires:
  Dfc_id_nv/1 -> Bit Clear2/1, Bit Set4/1, Bit Clear1/1
  Bit Set4/1 -> Bit Set/1
  Constant7/1 -> Delay2/1
  Delay2/1 -> Switch2/2
  Switch3/1 -> Switch2/3
  Bit Clear2/1 -> Switch2/1
  Switch2/1 -> Delay3/1, Switch1/1
  Bit Set1/1 -> Switch3/1
  Bit Set/1 -> Bit Set1/1
  Switch4/1 -> Switch3/3
  Err/1 -> Logical Operator/2, Switch3/2
  Bit Set2/1 -> Switch4/1
  Bit Clear1/1 -> Bit Set2/1
  Delay3/1 -> Switch4/3
  Heal/1 -> Logical Operator/1, Switch4/2
  Logical Operator/1 -> Switch1/2
  Constant1/1 -> Switch1/3
  Switch1/1 -> Dfc_id/1

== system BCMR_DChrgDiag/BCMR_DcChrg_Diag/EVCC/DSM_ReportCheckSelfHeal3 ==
  note: Fault report to diagnostic management system
  Dfc_id_nv : Inport  OutDataTypeStr=uint8
  Err : Inport  Port=2
  Heal : Inport  Port=3
  Bit Clear1 : simulink/Logic and Bit Operations/Bit Clear  iBit=4
  Bit Clear2 : simulink/Logic and Bit Operations/Bit Clear  iBit=3
  Bit Set : simulink/Logic and Bit Operations/Bit Set  iBit=4
  Bit Set1 : simulink/Logic and Bit Operations/Bit Set  iBit=3
  Bit Set2 : simulink/Logic and Bit Operations/Bit Set  iBit=3
  Bit Set4 : simulink/Logic and Bit Operations/Bit Set  iBit=7
  Constant1 : Constant  Value=0  OutDataTypeStr=uint8
  Constant7 : Constant  Value=0  OutDataTypeStr=boolean
  Delay2 : Delay  DelayLength=1  InitialCondition=1
  Delay3 : Delay  DelayLength=1  InitialCondition=0
  Logical Operator : Logic  Operator=OR  AllPortsSameDT=off  OutDataTypeStr=boolean
  Switch{1..4} (4 alike) : Switch  Criteria=u2 ~= 0
  Dfc_id : Outport  OutDataTypeStr=uint8
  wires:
  Switch1/1 -> Dfc_id/1
  Constant1/1 -> Switch1/3
  Logical Operator/1 -> Switch1/2
  Heal/1 -> Switch4/2, Logical Operator/1
  Delay3/1 -> Switch4/3
  Bit Clear1/1 -> Bit Set2/1
  Bit Set2/1 -> Switch4/1
  Err/1 -> Switch3/2, Logical Operator/2
  Switch4/1 -> Switch3/3
  Bit Set/1 -> Bit Set1/1
  Bit Set1/1 -> Switch3/1
  Switch2/1 -> Switch1/1, Delay3/1
  Bit Clear2/1 -> Switch2/1
  Switch3/1 -> Switch2/3
  Delay2/1 -> Switch2/2
  Constant7/1 -> Delay2/1
  Bit Set4/1 -> Bit Set/1
  Dfc_id_nv/1 -> Bit Clear1/1, Bit Set4/1, Bit Clear2/1

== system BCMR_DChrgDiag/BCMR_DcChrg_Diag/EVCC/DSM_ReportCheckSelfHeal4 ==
  note: Fault report to diagnostic management system
  Dfc_id_nv : Inport  OutDataTypeStr=uint8
  Err : Inport  Port=2
  Heal : Inport  Port=3
  Bit Clear1 : simulink/Logic and Bit Operations/Bit Clear  iBit=4
  Bit Clear2 : simulink/Logic and Bit Operations/Bit Clear  iBit=3
  Bit Set : simulink/Logic and Bit Operations/Bit Set  iBit=4
  Bit Set1 : simulink/Logic and Bit Operations/Bit Set  iBit=3
  Bit Set2 : simulink/Logic and Bit Operations/Bit Set  iBit=3
  Bit Set4 : simulink/Logic and Bit Operations/Bit Set  iBit=7
  Constant1 : Constant  Value=0  OutDataTypeStr=uint8
  Constant7 : Constant  Value=0  OutDataTypeStr=boolean
  Delay2 : Delay  DelayLength=1  InitialCondition=1
  Delay3 : Delay  DelayLength=1  InitialCondition=0
  Logical Operator : Logic  Operator=OR  AllPortsSameDT=off  OutDataTypeStr=boolean
  Switch{1..4} (4 alike) : Switch  Criteria=u2 ~= 0
  Dfc_id : Outport  OutDataTypeStr=uint8
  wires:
  Switch1/1 -> Dfc_id/1
  Constant1/1 -> Switch1/3
  Logical Operator/1 -> Switch1/2
  Heal/1 -> Switch4/2, Logical Operator/1
  Delay3/1 -> Switch4/3
  Bit Clear1/1 -> Bit Set2/1
  Bit Set2/1 -> Switch4/1
  Err/1 -> Switch3/2, Logical Operator/2
  Switch4/1 -> Switch3/3
  Bit Set/1 -> Bit Set1/1
  Bit Set1/1 -> Switch3/1
  Switch2/1 -> Switch1/1, Delay3/1
  Bit Clear2/1 -> Switch2/1
  Switch3/1 -> Switch2/3
  Delay2/1 -> Switch2/2
  Constant7/1 -> Delay2/1
  Bit Set4/1 -> Bit Set/1
  Dfc_id_nv/1 -> Bit Clear1/1, Bit Set4/1, Bit Clear2/1

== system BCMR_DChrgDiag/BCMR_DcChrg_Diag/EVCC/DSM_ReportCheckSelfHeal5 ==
  note: Fault report to diagnostic management system
  Dfc_id_nv : Inport  OutDataTypeStr=uint8
  Err : Inport  Port=2
  Heal : Inport  Port=3
  Bit Clear1 : simulink/Logic and Bit Operations/Bit Clear  iBit=4
  Bit Clear2 : simulink/Logic and Bit Operations/Bit Clear  iBit=3
  Bit Set : simulink/Logic and Bit Operations/Bit Set  iBit=4
  Bit Set1 : simulink/Logic and Bit Operations/Bit Set  iBit=3
  Bit Set2 : simulink/Logic and Bit Operations/Bit Set  iBit=3
  Bit Set4 : simulink/Logic and Bit Operations/Bit Set  iBit=7
  Constant1 : Constant  Value=0  OutDataTypeStr=uint8
  Constant7 : Constant  Value=0  OutDataTypeStr=boolean
  Delay2 : Delay  DelayLength=1  InitialCondition=1
  Delay3 : Delay  DelayLength=1  InitialCondition=0
  Logical Operator : Logic  Operator=OR  AllPortsSameDT=off  OutDataTypeStr=boolean
  Switch{1..4} (4 alike) : Switch  Criteria=u2 ~= 0
  Dfc_id : Outport  OutDataTypeStr=uint8
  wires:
  Dfc_id_nv/1 -> Bit Clear2/1, Bit Set4/1, Bit Clear1/1
  Bit Set4/1 -> Bit Set/1
  Constant7/1 -> Delay2/1
  Delay2/1 -> Switch2/2
  Switch3/1 -> Switch2/3
  Bit Clear2/1 -> Switch2/1
  Switch2/1 -> Delay3/1, Switch1/1
  Bit Set1/1 -> Switch3/1
  Bit Set/1 -> Bit Set1/1
  Switch4/1 -> Switch3/3
  Err/1 -> Logical Operator/2, Switch3/2
  Bit Set2/1 -> Switch4/1
  Bit Clear1/1 -> Bit Set2/1
  Delay3/1 -> Switch4/3
  Heal/1 -> Logical Operator/1, Switch4/2
  Logical Operator/1 -> Switch1/2
  Constant1/1 -> Switch1/3
  Switch1/1 -> Dfc_id/1

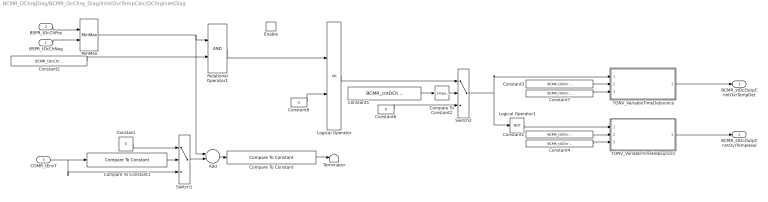
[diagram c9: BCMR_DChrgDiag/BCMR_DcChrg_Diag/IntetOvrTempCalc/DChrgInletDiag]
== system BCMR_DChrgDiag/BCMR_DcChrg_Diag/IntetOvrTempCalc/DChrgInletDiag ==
  BSPR_tDcChNeg : Inport
  BSPR_tDcChPos : Inport  Port=2
  COMR_tEnvT : Inport  Port=3
  Enable : EnablePort  StatesWhenEnabling=reset
  Add : Sum  Inputs=+-
  Compare To Constant : simulink/Logic and Bit Operations/Compare To Constant  relop=>=  const=BCMR_tDcChrgIntfTempDiffLmt_C  OutDataTypeStr=boolean
  Compare To Constant1 : simulink/Logic and Bit Operations/Compare To Constant  relop=<  const=BCMR_tiDChrgIntfTempDwnLmt_C  OutDataTypeStr=boolean
  Compare To Constant2 : simulink/Logic and Bit Operations/Compare To Constant  relop=~=  const=24  OutDataTypeStr=boolean
  Constant : Constant  Value=0
  Constant1 : Constant  Value=BCMR_tiDChrgDetDiagDebs_C
  Constant2 : Constant  Value=BCMR_tDcChrgIntfTempLmt_C  OutDataTypeStr=single
  Constant3 : Constant  Value=BCMR_tiDChrgDetDiagDebs_C
  Constant4 : Constant  Value=BCMR_tiDChrgDiagBase_C
  Constant5 : Constant  Value=BCMR_cntDChrgTCnntMax_C  OutDataTypeStr=single
  Constant6 : Constant  Value=0  OutDataTypeStr=boolean
  Constant7 : Constant  Value=BCMR_tiDChrgDiagBase_C
  Constant8 : Constant  Value=0  OutDataTypeStr=boolean
  Logical Operator : Logic  Operator=OR  AllPortsSameDT=off  OutDataTypeStr=boolean
  Logical Operator1 : Logic  Operator=NOT  AllPortsSameDT=off  OutDataTypeStr=boolean
  MinMax : MinMax  Function=max  Inputs=2
  Relational Operator1 : RelationalOperator  OutDataTypeStr=boolean  RndMeth=Simplest
  Switch1 : Switch  Criteria=u2 > Threshold
  Switch2 : Switch  Criteria=u2 > Threshold
  TONV_VariableTimeDebounce : Subsystem  TreatAsAtomicUnit=on  RTWFcnName=TONV_VariableTimeDebounce  RTWFileName=SrvLib
  TONV_VariableTimeDebounce1 : Subsystem  TreatAsAtomicUnit=on  RTWFcnName=TONV_VariableTimeDebounce  RTWFileName=SrvLib
  Terminator : Terminator
  BCMR_stDcOutpCnntOvrTempDet : Outport  OutputWhenDisabled=reset  InitialOutput=[0]
  BCMR_stDcOutpCnntOvrTempHeal : Outport  Port=2  OutputWhenDisabled=reset  InitialOutput=[1]
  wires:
  Compare To Constant1/1 -> Switch1/2
  Logical Operator/1 -> Switch2/1
  Add/1 -> Compare To Constant/1
  BSPR_tDcChPos/1 -> MinMax/1
  Constant2/1 -> Relational Operator1/2
  Relational Operator1/1 -> Logical Operator/1
  BSPR_tDcChNeg/1 -> MinMax/2
  COMR_tEnvT/1 -> Switch1/3, Compare To Constant1/1
  Switch1/1 -> Add/2
  Constant3/1 -> TONV_VariableTimeDebounce/2(T)
  Constant/1 -> Switch1/1
  MinMax/1 -> Add/1, Relational Operator1/1
  Constant8/1 -> Logical Operator/2
  Constant5/1 -> Compare To Constant2/1
  Logical Operator1/1 -> TONV_VariableTimeDebounce1/1(u)
  Constant4/1 -> TONV_VariableTimeDebounce1/3(dT)
  Switch2/1 -> TONV_VariableTimeDebounce/1(u), Logical Operator1/1
  Constant7/1 -> TONV_VariableTimeDebounce/3(dT)
  Compare To Constant2/1 -> Switch2/2
  Constant6/1 -> Switch2/3
  Compare To Constant/1 -> Terminator/1
  Constant1/1 -> TONV_VariableTimeDebounce1/2(T)
  TONV_VariableTimeDebounce/1(y) -> BCMR_stDcOutpCnntOvrTempDet/1
  TONV_VariableTimeDebounce1/1(y) -> BCMR_stDcOutpCnntOvrTempHeal/1

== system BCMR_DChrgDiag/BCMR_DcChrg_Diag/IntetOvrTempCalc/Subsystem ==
  BCMR_stDcOutpCnntOvrTempDet : Inport
  BCMR_stDcOutpCnntOvrTempHeal : Inport  Port=2
  Bitwise Operator1 : simulink/Logic and Bit Operations/Bitwise Operator  logicop=AND  UseBitMask=on  BitMask=bin2dec('00011000')  BitMaskRealWorld=Stored Integer
  Compare To Constant8 : simulink/Logic and Bit Operations/Compare To Constant  relop===  const=24  OutDataTypeStr=boolean
  DSM_ReportCheckSelfHeal : Subsystem  TreatAsAtomicUnit=on  RTWFcnName=DSM_ReportCheck  RTWFileName=SrvLib
  Data Store Read : DataStoreRead  DataStoreName=DFC_DChrgTCnntMax
  Data Store Read1 : DataStoreRead  DataStoreName=DFC_DChrgTCnntMax
  Data Store Write : DataStoreWrite  DataStoreName=DFC_DChrgTCnntMax
  Data Type Conversion : DataTypeConversion  OutDataTypeStr=uint8
  BCMR_stDcOutpCnntOvrTempErr : Outport  OutputWhenDisabled=reset  InitialOutput=[0]
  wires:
  DSM_ReportCheckSelfHeal/1(Dfc_id) -> Data Store Write/1
  Bitwise Operator1/1 -> Compare To Constant8/1
  Data Type Conversion/1 -> BCMR_stDcOutpCnntOvrTempErr/1  "BCMR_stDcOutpCnntOvrTempErr"
  Data Store Read/1 -> DSM_ReportCheckSelfHeal/1(Dfc_id_nv)
  Data Store Read1/1 -> Bitwise Operator1/1
  Compare To Constant8/1 -> Data Type Conversion/1
  BCMR_stDcOutpCnntOvrTempDet/1 -> DSM_ReportCheckSelfHeal/2(Err)
  BCMR_stDcOutpCnntOvrTempHeal/1 -> DSM_ReportCheckSelfHeal/3(Heal)

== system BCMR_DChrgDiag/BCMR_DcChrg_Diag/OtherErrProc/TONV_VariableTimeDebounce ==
  note: Turn On Delay Time Deboune
  u : Inport
  T : Inport  Port=2
  dT : Inport  Port=3
  Add : Sum
  Constant1 : Constant  Value=0  OutDataTypeStr=single
  Constant2 : Constant  OutDataTypeStr=uint8
  Constant3 : Constant  Value=0  OutDataTypeStr=uint8
  Delay : Delay  DelayLength=1  InitialCondition=0
  MinMax : MinMax  Inputs=2
  Product : Product  OutMin=[0]  OutMax=[65535]  OutDataTypeStr=single
  Relational Operator : RelationalOperator  Operator=>  OutDataTypeStr=boolean  RndMeth=Simplest
  Switch : Switch  Criteria=u2 ~= 0
  Switch1 : Switch  Criteria=u2 ~= 0
  y : Outport
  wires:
  Switch1/1 -> Product/1
  Constant3/1 -> Switch1/3
  Constant2/1 -> Switch1/1
  u/1 -> Switch1/2, Switch/2
  dT/1 -> Switch/1
  Constant1/1 -> Switch/3
  Add/1 -> Product/2
  Product/1 -> Relational Operator/1, Delay/1
  Switch/1 -> Add/1
  Delay/1 -> MinMax/2
  Relational Operator/1 -> y/1
  T/1 -> MinMax/1, Relational Operator/2
  MinMax/1 -> Add/2

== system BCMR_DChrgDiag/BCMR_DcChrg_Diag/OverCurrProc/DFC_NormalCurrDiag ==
  BCMR_bDcChrgCurrOutRngErrDet : Inport
  BCMR_bDcChrgCurrOutRngErrHeal : Inport  Port=2
  BCMR_bDcChrgOvrCurrErrDet : Inport  Port=3
  BCMR_bDcChrgOvrCurrErrHeal : Inport  Port=4
  BCMR_bDChrgCutOffVoltOvrCurrDet : Inport  Port=5
  BCMR_bDChrgCutOffVoltOvrCurrHeal : Inport  Port=6
  Bitwise Operator1 : simulink/Logic and Bit Operations/Bitwise Operator  logicop=AND  UseBitMask=on  BitMask=bin2dec('00011000')  BitMaskRealWorld=Stored Integer
  Compare To Constant8 : simulink/Logic and Bit Operations/Compare To Constant  relop===  const=24  OutDataTypeStr=boolean
  DSM_ReportCheckSelfHeal : Subsystem  TreatAsAtomicUnit=on  RTWFcnName=DSM_ReportCheck  RTWFileName=SrvLib
  Data Store Read : DataStoreRead  DataStoreName=DFC_DChrgCurrMish
  Data Store Read1 : DataStoreRead  DataStoreName=DFC_DChrgCurrMish
  Data Store Write : DataStoreWrite  DataStoreName=DFC_DChrgCurrMish
  Data Type Conversion1 : DataTypeConversion  OutDataTypeStr=uint8
  Logical Operator4 : Logic  Operator=OR  Inputs=3  AllPortsSameDT=off  OutDataTypeStr=boolean
  Logical Operator5 : Logic  Inputs=3  AllPortsSameDT=off  OutDataTypeStr=boolean
  BCMR_stBattNormalTempDChrgCurrOvrErr : Outport  OutputWhenDisabled=reset  InitialOutput=[0]
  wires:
  BCMR_bDcChrgCurrOutRngErrHeal/1 -> Logical Operator5/1
  BCMR_bDcChrgOvrCurrErrHeal/1 -> Logical Operator5/2
  BCMR_bDcChrgOvrCurrErrDet/1 -> Logical Operator4/2
  Data Type Conversion1/1 -> BCMR_stBattNormalTempDChrgCurrOvrErr/1  "BCMR_stBattNormalTempDChrgCurrOvrErr"
  Logical Operator5/1 -> DSM_ReportCheckSelfHeal/3(Heal)
  Logical Operator4/1 -> DSM_ReportCheckSelfHeal/2(Err)
  DSM_ReportCheckSelfHeal/1(Dfc_id) -> Data Store Write/1
  Data Store Read/1 -> DSM_ReportCheckSelfHeal/1(Dfc_id_nv)
  Compare To Constant8/1 -> Data Type Conversion1/1
  Bitwise Operator1/1 -> Compare To Constant8/1
  Data Store Read1/1 -> Bitwise Operator1/1
  BCMR_bDChrgCutOffVoltOvrCurrDet/1 -> Logical Operator4/3
  BCMR_bDChrgCutOffVoltOvrCurrHeal/1 -> Logical Operator5/3
  BCMR_bDcChrgCurrOutRngErrDet/1 -> Logical Operator4/1

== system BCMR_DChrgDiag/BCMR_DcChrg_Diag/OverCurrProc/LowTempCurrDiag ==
  BCMR_iDChrgBattCurrReqCalc : Inport
  BSPR_iBattCurr : Inport  Port=2
  BCMR_bDChrgWkup : Inport  Port=3
  Enable : EnablePort  StatesWhenEnabling=reset
  Abs3 : Abs
  Add1 : Sum  Inputs=+-
  Compare To Constant : simulink/Logic and Bit Operations/Compare To Constant  relop=>=  const=BCMR_iDcChrgLowTempOvrCurrCutOff_C  OutDataTypeStr=boolean
  Compare To Constant1 : simulink/Logic and Bit Operations/Compare To Constant  relop=<  const=BCMR_iDcChrgLowTempOvrCurrHeal_C  OutDataTypeStr=boolean
  Compare To Constant2 : simulink/Logic and Bit Operations/Compare To Constant  relop=>=  const=BCMR_iDcChrgLowTempDiffOvrCurrMody_C  OutDataTypeStr=boolean
  Constant1 : Constant  Value=BCMR_tiDChrgDiagBase_C
  Constant10 : Constant  Value=BCMR_tiDChrgLowTOvrCurrDet_C
  Constant13 : Constant  Value=BCMR_tiDChrgDiagBase_C
  Constant2 : Constant  Value=BCMR_tiDChrgDetDiagDebs_C
  Constant8 : Constant  Value=BCMR_tiDChrgLowTOvrCurrHeal_C
  Constant9 : Constant  Value=BCMR_tiDChrgDiagBase_C
  EdgeRising : Subsystem  TreatAsAtomicUnit=on  RTWFcnName=EdgeRising  RTWFileName=SrvLib
  LowTempOvrCurrCnt : Subsystem  TreatAsAtomicUnit=on
  TONV_VariableTimeDebounce : Subsystem  TreatAsAtomicUnit=on  RTWFcnName=TONV_VariableTimeDebounce  RTWFileName=SrvLib
  TONV_VariableTimeDebounce1 : Subsystem  TreatAsAtomicUnit=on  RTWFcnName=TONV_VariableTimeDebounce  RTWFileName=SrvLib
  TONV_VariableTimeDebounce2 : Subsystem  TreatAsAtomicUnit=on  RTWFcnName=TONV_VariableTimeDebounce  RTWFileName=SrvLib
  BCMR_bDChrgLowTempOvrCurrErrDet : Outport  OutputWhenDisabled=reset  InitialOutput=[0]
  BCMR_bDChrgLowTempOvrCurrErrHeal : Outport  Port=2  OutputWhenDisabled=reset  InitialOutput=[0]
  BCMR_bDChrgLowTempCurrModifyEna : Outport  Port=3
  BCMR_bDChrgCurrOvrCnt : Outport  Port=4  InitialOutput=[0]
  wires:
  TONV_VariableTimeDebounce1/1(y) -> BCMR_bDChrgLowTempOvrCurrErrDet/1  "BCMR_bDChrgLowTempOvrCurrErrDet"
  TONV_VariableTimeDebounce2/1(y) -> BCMR_bDChrgLowTempOvrCurrErrHeal/1  "BCMR_bDChrgLowTempOvrCurrErrHeal"
  Compare To Constant/1 -> TONV_VariableTimeDebounce1/1(u)
  BCMR_iDChrgBattCurrReqCalc/1 -> Add1/2
  Constant13/1 -> TONV_VariableTimeDebounce1/3(dT)
  Constant10/1 -> TONV_VariableTimeDebounce1/2(T)
  Constant8/1 -> TONV_VariableTimeDebounce2/2(T)
  Constant9/1 -> TONV_VariableTimeDebounce2/3(dT)
  Compare To Constant1/1 -> TONV_VariableTimeDebounce2/1(u)
  Compare To Constant2/1 -> TONV_VariableTimeDebounce/1(u)
  Constant1/1 -> TONV_VariableTimeDebounce/3(dT)
  Constant2/1 -> TONV_VariableTimeDebounce/2(T)
  TONV_VariableTimeDebounce/1(y) -> LowTempOvrCurrCnt/Trigger, BCMR_bDChrgLowTempCurrModifyEna/1  "BCMR_bDChrgCurrModifyEna"
  LowTempOvrCurrCnt/1(Out1) -> BCMR_bDChrgCurrOvrCnt/1
  BCMR_bDChrgWkup/1 -> EdgeRising/1(u)
  EdgeRising/1(y) -> LowTempOvrCurrCnt/1(Rst)
  BSPR_iBattCurr/1 -> Abs3/1
  Abs3/1 -> Add1/1
  Add1/1 -> Compare To Constant2/1, Compare To Constant/1, Compare To Constant1/1
